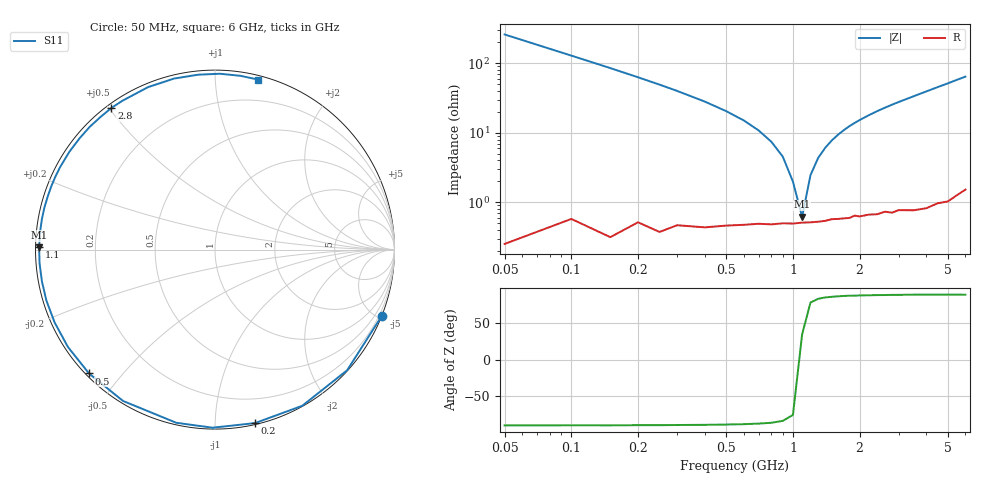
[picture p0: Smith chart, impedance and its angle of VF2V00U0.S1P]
! Infineon Technologies  Discrete & RF Semiconductors
! BBY 58-03
! Si Tuning Diode in SOD323
! VR = 2 V
! S-Parameters:  June  1999
# GHz  S  MA  R  50
!  f  S11
! GHz  MAG  ANG
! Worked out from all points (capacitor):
!   34 points, 50 MHz to 6 GHz, reference 50 ohm
!   read as one part to ground: C = 12.2 pF near 50 MHz
!   lowest |Z| = 618 mohm at 1.1 GHz (marker M1)
!   series resonance near 1.085 GHz, so ESL is about 1.8 nH
!   S11 on the Smith chart (normalised r, x): 50 MHz: 0.01, -5.19; 200 MHz: 0.01, -1.26; 500 MHz: 0.01, -0.41; 1.1 GHz: 0.01, +0.01; 2.8 GHz: 0.01, +0.51; 6 GHz: 0.03, +1.28
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0.05  0.9996 -21.8
0.1  0.997 -42.4
0.15  0.9968 -60.8
0.2  0.992 -77.0
0.25  0.9924 -90.8
0.3  0.9887 -102.6
0.4  0.9868 -121.3
0.5  0.9843 -135.5
0.6  0.9828 -146.5
0.7  0.9814 -155.6
0.8  0.9813 -163.2
0.9  0.9804 -169.7
1  0.9804 -175.6
1.1  0.9798 179.2
1.3  0.9794 170.1
1.6  0.978 158.7
1.8  0.9778 152.0
2  0.9774 146.1
2.2  0.9767 140.6
2.4  0.9772 135.5
2.8  0.9777 126.2
3  0.9767 122.0
3.5  0.979 112.4
4  0.9799 103.5
4.5  0.979 95.5
5  0.9802 88.4
5.5  0.9785 81.7
6  0.9773 75.8
